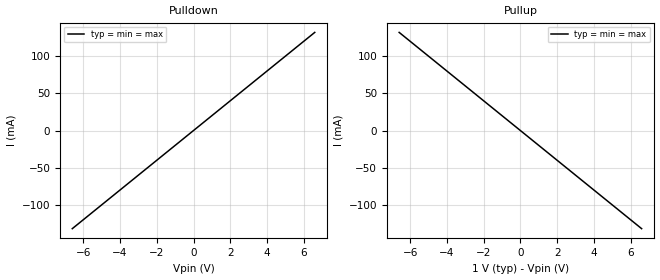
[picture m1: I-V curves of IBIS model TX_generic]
[IBIS Ver]   5.0
[File Name]   TX_generic.ibs
[File Rev]   1.0
[Component]   TX_generic
[Manufacturer] Texas Instruments
[Package]
R_pkg  0.0   NA   NA
L_pkg  0.0   NA   NA
C_pkg  0.0   NA   NA
[Pin]   signal_name   model_name   R_pin L_pin  C_pin
1p   TX_generic_p   TX_generic
1n   TX_generic_n   TX_generic
[Diff_Pin] inv_pin vdiff tdelay_typ tdelay_min tdelay_max
1p   1n   NA   NA   NA   NA
| Models and submodels in the file (1): TX_generic (Output)
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[Model] TX_generic
Model_type Output
C_comp 0p 0p 0p
Cref = 0
Vref = 0.5
Rref = 50
Vmeas = 0.5
[Temperature_Range] 25 125 0
[Voltage Range] 1.0 1.0 1.0
[Algorithmic Model]
Executable Windows_cl16.00.30319.01_64 TX_generic_x64.dll TX_generic.ami
Executable Windows_cl16.00.30319.01_32 TX_generic.dll TX_generic.ami
[End Algorithmic Model]
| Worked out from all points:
|   slope of the pulldown table from 0 to 0.15 V, typ, clamps not added: 50 ohm
|   slope of the pullup table from 0 to 0.15 V, typ, clamps not added: 50 ohm
[Pulldown]
-6.6V     -132mA     -132mA     -132mA
0V        0A         0A         0A
6.6V      132mA      132mA      132mA
[Pullup]
-6.6V     132mA      132mA      132mA
0V        0A         0A         0A
6.6V      -132mA     -132mA     -132mA
[GND Clamp]
-6.6V     0A         0A         0A
0V        0A         0A         0A
6.6V      0A         0A         0A
[Power Clamp]
-6.6V     0A         0A         0A
0V        0A         0A         0A
6.6V      0A         0A         0A
[Ramp]
|dV/dt_r 0.3/1.5p 0.3/1.5p 0.3/1.5p
|dV/dt_f 0.3/1.5p 0.3/1.5p 0.3/1.5p
dV/dt_r 0.3/20p 0.3/20p 0.3/20p
dV/dt_f 0.3/20p 0.3/20p 0.3/20p
